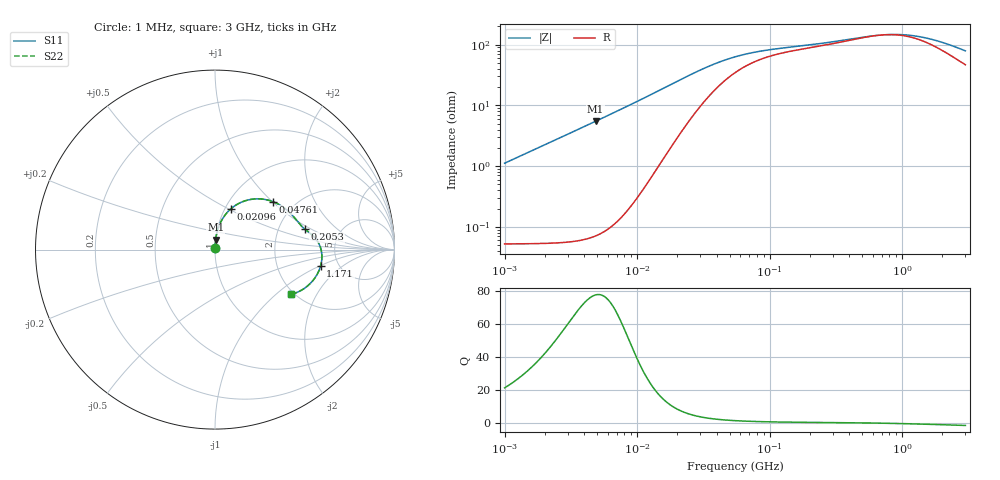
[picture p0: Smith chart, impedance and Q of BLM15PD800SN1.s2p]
! BLM15PD800SN1
# Hz S RI R 50
!Freq.(Hz) S11(Real) S11(Imag) S21(Real) S21(Imag) S12(Real) S12(Imag) S22(Real) S22(Imag)
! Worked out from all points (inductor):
!   401 points, 1 MHz to 3 GHz, reference 50 ohm
!   read as one part in series: L = 177 nH near 1.041 MHz
!   highest Q = 77.4 at 4.861 MHz (marker M1), where L = 179 nH
!   self-resonance near 712.5 MHz
!   S11 on the Smith chart (normalised r, x): 1 MHz: 1.00, +0.02; 20.96 MHz: 1.07, +0.52; 47.61 MHz: 1.55, +1.00; 205.3 MHz: 2.79, +0.87; 1.171 GHz: 3.65, -1.01; 3 GHz: 1.93, -1.27
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1000000  0.000646 0.0111  0.9994 -0.0111  0.9994 -0.0111  0.000646 0.0111
3823119  0.00243 0.0427  0.9976 -0.0427  0.9976 -0.0427  0.00243 0.0427
4861065  0.00368 0.0545  0.9963 -0.0545  0.9963 -0.0545  0.00368 0.0545
8686058  0.0118 0.0985  0.9882 -0.0985  0.9882 -0.0985  0.0118 0.0985
1.461624e7  0.0389 0.1664  0.9611 -0.1664  0.9611 -0.1664  0.0389 0.1664
2.095589e7  0.0895 0.228  0.9105 -0.228  0.9105 -0.228  0.0895 0.228
3.190472e7  0.1999 0.2798  0.8001 -0.2798  0.8001 -0.2798  0.1999 0.2798
3.897472e7  0.2626 0.2816  0.7374 -0.2816  0.7374 -0.2816  0.2626 0.2816
4.761141e7  0.3204 0.268  0.6796 -0.268  0.6796 -0.268  0.3204 0.268
5.477226e7  0.3549 0.2522  0.6451 -0.2522  0.6451 -0.2522  0.3549 0.2522
6.964249e7  0.4011 0.2201  0.5989 -0.2201  0.5989 -0.2201  0.4011 0.2201
9.034013e7  0.4356 0.186  0.5644 -0.186  0.5644 -0.186  0.4356 0.186
1.321429e8  0.4686 0.1464  0.5314 -0.1464  0.5314 -0.1464  0.4686 0.1464
2.052512e8  0.4988 0.1155  0.5012 -0.1155  0.5012 -0.1155  0.4988 0.1155
2.094008e8  0.5002 0.1144  0.4998 -0.1144  0.4998 -0.1144  0.5002 0.1144
4.391493e8  0.5599 0.0625  0.4401 -0.0625  0.4401 -0.0625  0.5599 0.0625
8.005644e8  0.5944 -0.0191  0.4056 0.0191  0.4056 0.0191  0.5944 -0.0191
1.171007e9  0.589 -0.0892  0.411 0.0892  0.411 0.0892  0.589 -0.0892
1.488926e9  0.5696 -0.1372  0.4304 0.1372  0.4304 0.1372  0.5696 -0.1372
1.855641e9  0.5387 -0.1803  0.4613 0.1803  0.4613 0.1803  0.5387 -0.1803
2.407135e9  0.4847 -0.2244  0.5153 0.2244  0.5153 0.2244  0.4847 -0.2244
3e9  0.4261 -0.2492  0.5739 0.2492  0.5739 0.2492  0.4261 -0.2492
